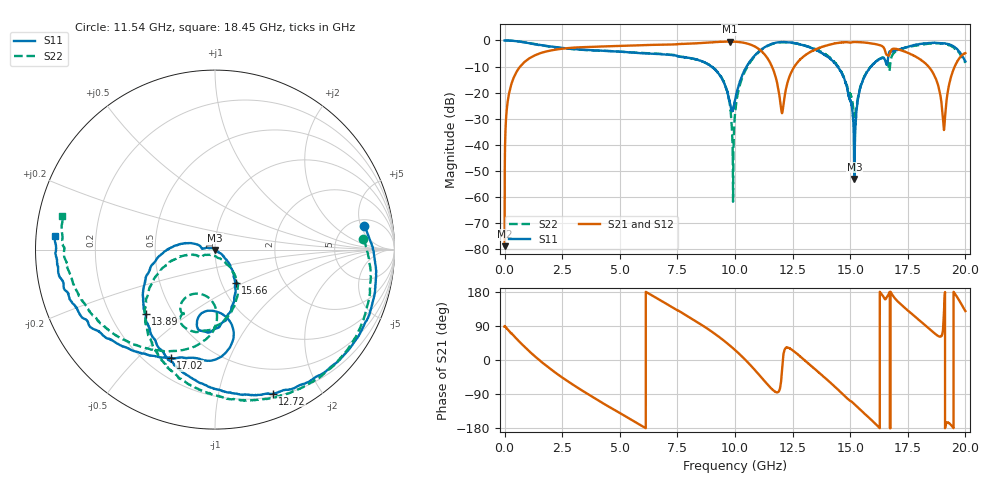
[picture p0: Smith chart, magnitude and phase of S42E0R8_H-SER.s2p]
!{S42E0R8}
!Johanson Technology Inc.
!www.johansontechnology.com
!Test Board Conditions:
!Substrate Type  RO4350B
!Substrate Thickness  50 mil
!Substrate Dk  3.66
!TL Type: GCPW
!TL Trace Width  60 mil
!TL Gap  10 mil
!Electrode orientation  Horizontal
!DUT TOPOLOGY	SERIES
!Mounting Pad LxW  14x55 mil
! Created Wed Nov 25 21:28:16 2020
# khz S ma R 50
! 2 Port Network Data from SP1.SP block
! freq  magS11  angS11  magS21  angS21  magS12  angS12  magS22  angS22
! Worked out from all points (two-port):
!   20001 points, 300 kHz to 20 GHz, reference 50 ohm
!   highest |S21| = -0.42 dB at 9.765 GHz (marker M1); lowest = -78.8 dB at 300 kHz (marker M2)
!   |S21| within 3 dB of the highest: 2.287 GHz to 11.05 GHz (8.764 GHz wide, 131 % of centre); 13.5 GHz to 16.49 GHz (2.996 GHz wide, 20 % of centre)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
!   lowest |S11| = -53.0 dB at 15.19 GHz (marker M3), VSWR 1.00, Z = 50 - j0.223 ohm
!   |S11| at or under -10 dB: 8.976891 GHz to 8.977495 GHz (604.2 kHz wide, 0.00673 % of centre); 8.979 GHz to 10.5 GHz (1.526 GHz wide, 15.7 % of centre); 14.45 GHz to 15.91 GHz (1.456 GHz wide, 9.59 % of centre)
!   |S22| runs from -61.8 to 0.0 dB; largest |S21 - S12| = 0.018
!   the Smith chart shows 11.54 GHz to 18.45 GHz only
!   S11 on the Smith chart (normalised r, x): 11.54 GHz: 6.30, +5.75; 12.72 GHz: 0.23, -1.45; 13.89 GHz: 0.35, -0.35; 15.66 GHz: 1.16, -0.45; 17.02 GHz: 0.30, -0.63; 18.45 GHz: 0.06, +0.04
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300  0.9995 -0.2  0.000115 87.7  0.0001748 103.1  0.9993 -0.3
129300  0.9972 -8.5  0.06501 81.1  0.06523 81.0  0.9976 -8.6
499300  0.9694 -32.7  0.2416 57.3  0.2423 57.5  0.9694 -32.8
3334300  0.6666 -170.9  0.7412 -79.4  0.741 -79.4  0.6627 -168.0
6667300  0.5494 77.9  0.8272 160.8  0.8253 160.7  0.5558 64.9
8970300  0.3176 -16.4  0.9182 75.7  0.9197 75.8  0.3203 -11.4
9765300  0.06866 -20.9  0.9528 38.8  0.953 38.9  0.06427 -49.2
1.00003e7  0.07112 66.6  0.9448 26.4  0.9447 26.5  0.03912 121.9
1.04043e7  0.2637 75.1  0.8999 3.2  0.8982 3.3  0.2413 92.5
1.15353e7  0.8415 9.1  0.3663 -72.6  0.3649 -72.1  0.8289 4.2
1.20433e7  0.9315 -25.4  0.04094 -23.8  0.04138 -24.1  0.9234 -34.8
1.27243e7  0.8644 -68.2  0.3854 14.8  0.3924 14.3  0.8619 -77.3
1.33343e7  0.7114 -104.0  0.6217 -17.1  0.6214 -17.5  0.7215 -108.7
1.38933e7  0.5276 -136.9  0.7819 -46.4  0.7742 -46.7  0.5565 -134.2
1.47093e7  0.2008 171.2  0.9222 -91.7  0.9198 -91.6  0.2049 -168.3
1.51863e7  0.002227 -91.6  0.9375 -116.8  0.9398 -117.0  0.03504 -108.7
1.56563e7  0.2177 -58.3  0.9055 -143.5  0.9143 -143.3  0.2221 -56.3
1.66673e7  0.5326 -80.0  0.5136 173.3  0.5059 172.9  0.3141 -121.5
1.70213e7  0.6516 -112.3  0.6844 157.2  0.6717 157.2  0.6337 -116.5
1.84483e7  0.8924 175.1  0.2976 81.4  0.2994 82.1  0.8728 167.5
1.90723e7  0.8796 135.9  0.0193 131.4  0.01958 131.2  0.8595 132.8
2e7  0.3941 64.7  0.572 129.1  0.5754 129.4  0.3726 80.0
